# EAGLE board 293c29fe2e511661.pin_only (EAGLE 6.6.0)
REV: D

Size 50.8 x 22.86 mm. Coordinates in mm from the lower left corner, seen from the top.
Outline: 2.54,0 48.26,0 arc90 50.8,2.54 50.8,20.32 arc90 48.26,22.86 2.54,22.86 arc90 0,20.32 0,13.84 0.51,13.34 0.51,9.53 0,9.02 0,2.54 arc90 2.54,0
Copper layers (1*16): Top 0.035mm / dielectric 1.5mm / Bottom 0.035mm
Design rules "adafruit *": minimum track width 8mil, minimum drill 15.5mil, track to track 8mil, track to pad 8mil, pad to pad 8mil, via to via 8mil, smd to smd 8mil, copper to edge 10mil, drill to drill 8mil, minimum pad ring 10mil, minimum via ring 8mil, stop-mask expansion 2mil, vias tented up to drill 20mil, thermal gap 10mil
tRestrict: area 23.4,8.3 to 26.5,8.6; area 26.2,8.4 to 26.7,9.9; area 21.2,13.6 to 25.9,14.1; area 20.8,13.3 to 21.2,13.7; area 20.7,9.3 to 21.2,13; area 20.7,8.1 to 21.2,8.9; area 21.1,8.1 to 23,8.6; area 26.2,10.3 to 26.7,13.3

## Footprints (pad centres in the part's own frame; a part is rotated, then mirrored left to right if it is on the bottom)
0603-NO = smd 1.1 x 1: 1 -0.85,0; 2 0.85,0
0805-NO = smd 1.3 x 1.5: 1 -0.95,0; 2 0.95,0
_0805MP = smd 1.2 x 1.3: 1 -1.016,0; 2 1.016,0
CHIPLED_0805_NOOUTLINE = smd 1.2 x 1.2: A 0,-1.05; C 0,1.05
SOD-123 = smd 1.4 x 1.4: A 1.85,0; C -1.85,0
TQFN44_7MM = smd 0.25 x 0.8: 1 -2.5,-3.475; 2 -2,-3.475; 3 -1.5,-3.475; 4 -1,-3.475; 5 -0.5,-3.475; 6 0,-3.475; 7 0.5,-3.475; 8 1,-3.475; 9 1.5,-3.475; 10 2,-3.475; 11 2.5,-3.475; 23 2.5,3.475; 24 2,3.475; 25 1.5,3.475; 26 1,3.475; 27 0.5,3.475; 28 0,3.475; 29 -0.5,3.475; 30 -1,3.475; 31 -1.5,3.475; 32 -2,3.475; 33 -2.5,3.475 | smd 0.8 x 0.25: 12 3.475,-2.5; 13 3.475,-2; 14 3.475,-1.5; 15 3.475,-1; 16 3.475,-0.5; 17 3.475,0; 18 3.475,0.5; 19 3.475,1; 20 3.475,1.5; 21 3.475,2; 22 3.475,2.5; 34 -3.475,2.5; 35 -3.475,2; 36 -3.475,1.5; 37 -3.475,1; 38 -3.475,0.5; 39 -3.475,0; 40 -3.475,-0.5; 41 -3.475,-1; 42 -3.475,-1.5; 43 -3.475,-2; 44 -3.475,-2.5 | smd 4.7 x 4.7: THERMAL 0,0
1X16_ROUND = drill 1 pad 1.676: 1 -19.05,0; 2 -16.51,0; 3 -13.97,0; 4 -11.43,0; 5 -8.89,0; 6 -6.35,0; 7 -3.81,0; 8 -1.27,0; 9 1.27,0; 10 3.81,0; 11 6.35,0; 12 8.89,0; 13 11.43,0; 14 13.97,0; 15 16.51,0; 16 19.05,0
1X12_ROUND = drill 1 pad 1.676: 1 -13.97,0; 2 -11.43,0; 3 -8.89,0; 4 -6.35,0; 5 -3.81,0; 6 -1.27,0; 7 1.27,0; 8 3.81,0; 9 6.35,0; 10 8.89,0; 11 11.43,0; 12 13.97,0
KMR2 = smd 1 x 1: 1 2,0.8; 2 2,-0.8; 3 -2,0.8; 4 -2,-0.8
PAD-1.5X2.0 = smd 1.5 x 2: P$1 0,0
BLE_MODULE_RAYTAC_MDBT40 = smd 1.85 x 0.45: 1 -4.825,4; 2 -4.825,3.3; 3 -4.825,-0.9; 4 -4.825,-1.6; 5 -4.825,-2.3; 6 -4.825,-3; 7 -4.825,-3.7; 8 -4.825,-4.4; 9 -4.825,-5.1; 10 -4.825,-5.8; 11 -4.825,-6.5; 12 -4.825,-7.2; 26 4.825,-7.2; 27 4.825,-6.5; 28 4.825,-5.8; 29 4.825,-5.1; 30 4.825,-4.4; 31 4.825,-3.7; 32 4.825,-3; 33 4.825,-2.3; 34 4.825,-1.6; 35 4.825,-0.9; 36 4.825,-0.2; 37 4.825,0.5; 38 4.825,1.2; 39 4.825,1.9; 40 4.825,2.6; 41 4.825,3.3; 42 4.825,4 | smd 0.45 x 1.85: 13 -4.2,-8.825; 14 -3.5,-8.825; 15 -2.8,-8.825; 16 -2.1,-8.825; 17 -1.4,-8.825; 18 -0.7,-8.825; 19 0,-8.825; 20 0.7,-8.825; 21 1.4,-8.825; 22 2.1,-8.825; 23 2.8,-8.825; 24 3.5,-8.825; 25 4.2,-8.825 | hole 0.9: 2.2,4.45
SOT23-5 = smd 0.55 x 1.2: 1 -0.95,-1.3; 2 0,-1.3; 3 0.95,-1.3; 4 0.95,1.3; 5 -0.95,1.3
MOUNTINGHOLE_2.5_PLATED = drill 2.5 pad 3.2: P$1 0,0
FIDUCIAL_1MM = smd 1 x 1: 1 0,0
JSTPH2 = smd 1 x 4.6: 1 -1,-3.7; 2 1,-3.7 | smd 1.6 x 3.4: NC1 -3.4,1.5; NC2 3.4,1.5
4UCONN_20329_V2 = smd 1 x 2: BASE@1 -0.75,-2; BASE@2 0.75,-2 | smd 0.4 x 1.35: D+ 0,0.775; D- -0.65,0.775; GND 1.3,0.775; ID 0.65,0.775; VBUS -1.3,0.775 | drill 0.8 pad 1.2 offset: SPRT@1 -3.3,0.9; SPRT@2 3.3,0.9 | drill 0.9 pad 2.5 square: SPRT@3 -3.6,-1.9; SPRT@4 3.6,-1.9 | hole 0.7: -1.95,0; 1.95,0
RESONATOR-SMD = smd 0.7 x 1.7: 1 -1.2,0; 2 0,0; 3 1.2,0

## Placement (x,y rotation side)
C2  1uF  [0603-NO]  41.02,18.41 0 top
C3  10µF  [0805-NO]  11.81,12.06 0 top
C6  10µF  [0805-NO]  8.09,12.96 90 top
C7  1uF  [0603-NO]  19.07,15.04 90 top
C8  10µF  [0805-NO]  14.37,11.37 270 top
C9  10uF  [_0805MP]  29.57,14.83 180 top
C14  1uF  [0603-NO]  10.34,4.09 0 top
CHG  ORANGE  [CHIPLED_0805_NOOUTLINE]  2.41,5.59 270 top
D1  RED  [CHIPLED_0805_NOOUTLINE]  48.64,17.4 270 top
D2  BLUE  [CHIPLED_0805_NOOUTLINE]  48.51,5.33 270 top
D4  MBR120  [SOD-123]  17.91,18.92 180 top
IC1  ATMEGA32U4-MU  [TQFN44_7MM]  23.72,11.1 0 top
JP1  [1X16_ROUND]  25.4,1.27 180 top
JP3  [1X12_ROUND]  30.48,21.59 0 top
L  RED  [CHIPLED_0805_NOOUTLINE]  2.65,17.36 90 top
R1  2.2K  [0603-NO]  44.32,18.41 0 top
R2  1K  [0603-NO]  6.22,4.19 0 top
R3  100K  [0603-NO]  30.23,17.78 0 top
R4  22  [0603-NO]  8.22,10.27 0 top
R5  22  [0603-NO]  8.15,8.88 0 top
R6  100K  [0603-NO]  31.62,19.05 0 top
R7  2.2K  [0603-NO]  5.59,20.95 270 top
R8  10K\  [0603-NO]  13.84,4.06 180 top
R9  100K  [0603-NO]  17.4,17.42 180 top
R10  2.2K  [0603-NO]  44.45,4.57 0 top
SW1  SPST_TACT-KMR2  [KMR2]  9.4,6.48 180 top
TP1  SWCLK  [PAD-1.5X2.0]  43.05,9.53 0 bottom
TP2  SWDIO  [PAD-1.5X2.0]  40.77,9.53 0 bottom
TP3  SWDIO  [PAD-1.5X2.0]  38.48,9.53 0 bottom
U1  MBT40  [BLE_MODULE_RAYTAC_MDBT40]  41.66,11.43 270 top
U2  SPX3819-3.3  [SOT23-5]  16.56,14.81 180 top
U3  MCP73831T-2ACI/OT  [SOT23-5]  13.97,7.49 180 top
U$6  MOUNTINGHOLE2.5  [MOUNTINGHOLE_2.5_PLATED]  48.26,20.32 0 top
U$7  [ADAFRUIT_3.5MM]  15.88,8.26 0 top
U$9  [FEATHERLOGO]  37.47,5.59 0 bottom
U$23  [PCBFEAT-REV-040]  1.27,17.53 0 bottom
U$24  MOUNTINGHOLE2.5  [MOUNTINGHOLE_2.5_PLATED]  48.26,2.54 0 top
U$26  [BLUEFRUITLOGO_100MM]  13.97,7.49 0 bottom
U$31  MOUNTINGHOLE2.5  [MOUNTINGHOLE_2.5_PLATED]  2.54,20.32 270 top
U$32  MOUNTINGHOLE2.5  [MOUNTINGHOLE_2.5_PLATED]  2.54,2.54 270 top
U$34  FIDUCIAL""  [FIDUCIAL_1MM]  10.79,20.07 270 top
U$35  FIDUCIAL""  [FIDUCIAL_1MM]  45.39,13.98 270 top
X1  JSTPH  [JSTPH2]  10.67,19.3 0 top
X3  microUSB  [4UCONN_20329_V2]  4.45,11.43 270 top
Y1  8MHz  [RESONATOR-SMD]  28.25,5.26 180 top

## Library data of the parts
C2 C3 C6 C7 C9 C14 CHG D1 D2 D4 IC1 JP1 JP3 L R1-R10 TP1-TP3 U1-U3 U$7 U$9 U$23 X1 X3 = microbuilder
C8 = microbuilder; COMPANY: ADAFRUIT INDUSTRIES; DRAWN: KTOWN; REV: A
SW1 U$26 = adafruit
U$6 U$31 U$32 U$34 U$35 = microbuilder; BOM: EXCLUDE
U$24 = microbuilder; BOM: EXCLUDE; COMPANY: ADAFRUIT INDUSTRIES; DRAWN: KTOWN; REV: A
Y1 = SparkFun

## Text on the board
tPlace: 3 | 2 | BAT | En | USB | 13 | 12 | 11 | ~ | 10 | 9 | 6 | ~5 | SCL | SDA | ~ | #13 | ~ | Feather / Bluefruit | 32u4 | adafruit! | RST | CHG | RX | TX | A3 | A4 | A5 | SCK | MOSI | MISO | RST | 3V | ARf | GND | A0 | A1 | A2 | 0 | 1 | DFU
bPlace: 3 | 2 | 3.7/4.2V / LiPoly Batt / µUSB charge | 6 | ~ | 5 | SCL | SDA | BAT | En | USB | 13 | 12 | 11~ | 10~ | 9~ | Feather 32u4 / Bluefruit LE | Bluefruit LE Pins: | SPI (SCK,MOSI,MISO) | ATmega32u4 / 8MHz & 3.3V | 4 Reset,7 IRQ,8 CS | Reset | SWDIO | SWCLK | MOSI | MISO | RST | 3V | Ref | GND | A0 | A1 | A2 | A3 | A4 | A5 | SCK | RX | TX | GND | 0 | 1

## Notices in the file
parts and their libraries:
microbuilder: This work is placed in the public domain, and may be freely used for commercial and non-commercial work with the following conditions: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
SparkFun: Licensing: CC v3.0 Share-Alike You are welcome to use this library for commercial purposes.
